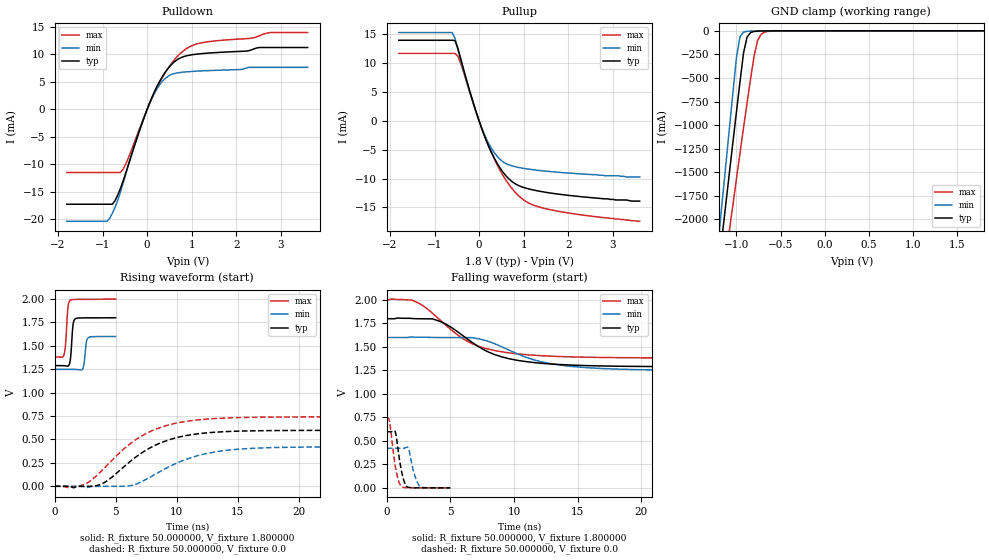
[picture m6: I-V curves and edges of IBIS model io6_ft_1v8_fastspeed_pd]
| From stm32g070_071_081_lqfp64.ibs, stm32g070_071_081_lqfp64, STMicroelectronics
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|   Model io6_ft_1v8_fastspeed_pd
[Model]  io6_ft_1v8_fastspeed_pd
Model_type I/O
Polarity   Non-Inverting
Enable   Active-Low
Vinl =   0.540000V
Vinh =   1.260000V
Vmeas =  0.900000V
Cref =   50.000000pF
Rref =   100.000000M
Vref =   0.0V
C_comp   1.277600pF   1.236700pF   1.315100pF
[Temperature Range]   25.000000   -40.000000   0.125000k
[Pullup Reference]   1.800000V   1.600000V   2.000000V
[Pulldown Reference]   0.0V   0.0V   0.0V
[POWER Clamp Reference]   1.800000V   1.600000V   2.000000V
[GND Clamp Reference]   0.0V   0.0V   0.0V
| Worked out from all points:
|   slope of the pulldown table from 0 to 0.27 V, typ, clamps not added: 54.7 ohm
|   slope of the pullup table from 0 to 0.27 V, typ, clamps not added: 50.6 ohm
|   GND clamp passes 1 mA (typ) near -0.66 V on its own axis
|   rising waveform, R_fixture 50.000000, V_fixture 1.800000: 20-80 % time 165ps typ, 169ps min, 180ps max; typ from 1.29 V to 1.8 V
|   rising waveform, R_fixture 50.000000, V_fixture 0.0: 20-80 % time 4.08ns typ, 4.39ns min, 4.26ns max; typ from 0 V to 0.597 V
|   falling waveform, R_fixture 50.000000, V_fixture 1.800000: 20-80 % time 3.95ns typ, 4.46ns min, 3.82ns max; typ from 1.8 V to 1.29 V
|   falling waveform, R_fixture 50.000000, V_fixture 0.0: 20-80 % time 436ps typ, 477ps min, 449ps max; typ from 0.597 V to 0 V
[Pulldown]
|Voltage   I(typ)   I(min)   I(max)
-1.8V     -17.22mA   -20.33mA   -11.45mA
-900mV    -17.22mA   -20.33mA   -11.45mA
-720mV    -16.58mA   -17.82mA   -11.45mA
-600mV    -14.41mA   -15.08mA   -11.45mA
-480mV    -11.58mA   -11.79mA   -9.954mA
0V        10fA       0A         100fA
240mV     4.49mA     3.999mA    4.291mA
480mV     7.563mA    6.085mA    7.612mA
780mV     9.487mA    6.76mA     10.43mA
1.14V     10.08mA    6.976mA    11.96mA
2.76V     11.26mA    7.652mA    13.98mA
3.6V      11.26mA    7.652mA    13.98mA
[Pullup]
|Voltage   I(typ)   I(min)   I(max)
-1.8V     14mA       15.33mA    11.72mA
-600mV    14mA       15.33mA    11.72mA
-540mV    13.93mA    14.32mA    11.72mA
-420mV    11.01mA    10.78mA    10.14mA
-180mV    4.421mA    4.232mA    4.225mA
60mV      -1.349mA   -1.244mA   -1.314mA
300mV     -5.831mA   -5.038mA   -5.917mA
600mV     -9.499mA   -7.385mA   -10.25mA
960mV     -11.43mA   -8.172mA   -13.47mA
1.32V     -12.13mA   -8.557mA   -14.86mA
2.16V     -13.03mA   -9.116mA   -16.14mA
3.6V      -13.9mA    -9.7mA     -17.4mA
[GND_clamp]
|Voltage   I(typ)   I(min)   I(max)
-1.8V     -7.471A    -7.973A    -7.298A
-1.2V     -2.489A    -2.18A     -2.954A
-1.16V    -2.16A     -1.797A    -2.674A
-1.08V    -1.505A    -1.034A    -2.118A
-1V       -858mA     -283.1mA   -1.568A
-960mV    -540.4mA   -62.15mA   -1.296A
-920mV    -234.4mA   -13.76mA   -1.028A
-880mV    -66.3mA    -4.868mA   -765.3mA
-800mV    -6.518mA   -2.068mA   -266mA
-760mV    -3.087mA   -1.462mA   -100.4mA
-680mV    -1.228mA   -569.1uA   -14.21mA
1.8V      47.47uA    34.04uA    59.57uA
[POWER_clamp]
|Voltage   I(typ)   I(min)   I(max)
-1.8V     0A         0A         0A
0V        0A         0A         0A
[Ramp]
| variable   typ   min   max
dV/dt_r  0.35813/4.07174n   0.25245/4.38021n   0.44110/4.25256n
dV/dt_f  0.30642/3.93587n   0.21030/4.44000n   0.37044/3.81917n
R_load = 50.000000
[Rising Waveform]
R_fixture= 50.000000
V_fixture= 1.800000
V_fixture_min= 1.600000
V_fixture_max= 2.000000
|time   V(typ)   V(min)   V(max)
0s        1.288V     1.248V     1.381V
770.8ps   1.287V     1.248V     1.411V
880.9ps   1.285V     1.248V     1.513V
1.081ns   1.284V     1.248V     1.91V
1.241ns   1.327V     1.248V     1.982V
1.491ns   1.72V      1.248V     1.994V
1.662ns   1.786V     1.248V     1.995V
2.302ns   1.798V     1.259V     1.996V
2.713ns   1.798V     1.582V     1.996V
4.985ns   1.799V     1.599V     1.998V
[Rising Waveform]
R_fixture= 50.000000
V_fixture= 0.0
V_fixture_min= 0.0
V_fixture_max= 0.0
|time   V(typ)   V(min)   V(max)
0s        -1.303uV   809.4nV    108.6nV
1.141ns   -1.02mV    -3.84uV    -16.89mV
2.222ns   -948.5uV   -326.3uV   10.6mV
3.664ns   15.82mV    -604.3uV   142.4mV
6.787ns   326.1mV    29.64mV    510.2mV
8.649ns   462.9mV    159mV      627.8mV
10.21ns   526.4mV    259.5mV    680.8mV
12.31ns   568.6mV    346.3mV    715.8mV
15.08ns   588.6mV    396.5mV    733.1mV
29.91ns   597.1mV    420.8mV    741.3mV
[Falling Waveform]
R_fixture= 50.000000
V_fixture= 1.800000
V_fixture_min= 1.600000
V_fixture_max= 2.000000
|time   V(typ)   V(min)   V(max)
0s        1.799V     1.599V     1.998V
2.042ns   1.801V     1.604V     1.993V
3.664ns   1.794V     1.6V       1.849V
4.745ns   1.733V     1.598V     1.717V
6.186ns   1.598V     1.598V     1.57V
7.568ns   1.474V     1.574V     1.491V
9.009ns   1.394V     1.502V     1.447V
11.47ns   1.334V     1.365V     1.412V
14.53ns   1.306V     1.291V     1.393V
29.91ns   1.288V     1.248V     1.381V
[Falling Waveform]
R_fixture= 50.000000
V_fixture= 0.0
V_fixture_min= 0.0
V_fixture_max= 0.0
|time   V(typ)   V(min)   V(max)
0s        597.1mV    420.8mV    741.3mV
230.2ps   596.6mV    420.9mV    693.5mV
660.7ps   597.3mV    421mV      237.1mV
870.9ps   423.6mV    421mV      96.77mV
1.101ns   217mV      420.5mV    22.46mV
1.381ns   61.14mV    422mV      3.655mV
1.682ns   5.993mV    425.9mV    1.469mV
2.192ns   926.9uV    135.8mV    801.5uV
2.653ns   283.7uV    9.933mV    577.3uV
4.985ns   -1.303uV   809.4nV    108.6nV
